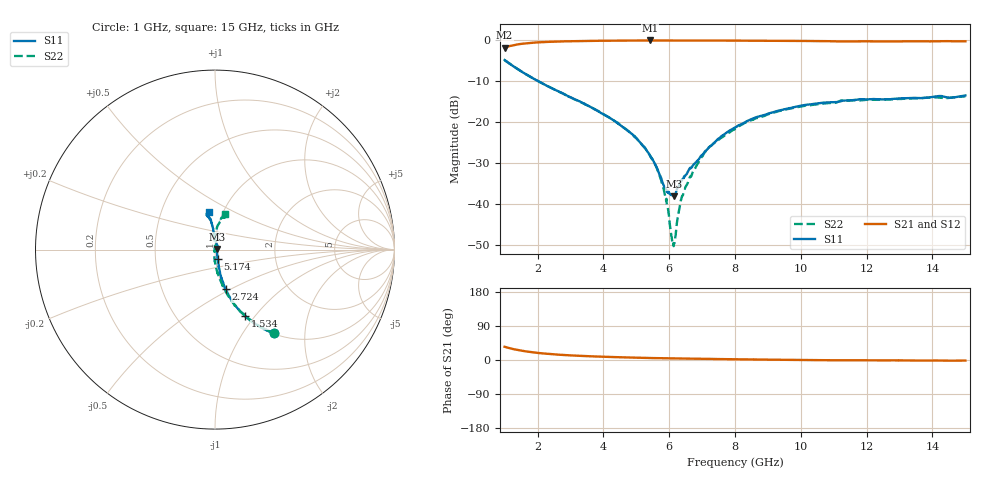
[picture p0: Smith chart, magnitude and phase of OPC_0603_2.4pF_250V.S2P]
! FILE NAME
! DATE 08/15/2012  09:51
! CORRECTED  DATA
# GHz  S  MA  R  50.00
!  FREQ  S11M  S11A  S21M  S21A  S12M  S12A  S22M  S22A
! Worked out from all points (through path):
!   1601 points, 1 GHz to 15 GHz, reference 50 ohm
!   highest |S21| = -0.06 dB at 5.419 GHz (marker M1); lowest = -1.8 dB at 1 GHz (marker M2)
!   group delay of S21, straight-line fit = 4.46 ps
!   lowest |S11| = -38.2 dB at 6.154 GHz (marker M3), VSWR 1.02, Z = 51.2 + j0.338 ohm
!   |S11| at or under -10 dB: 2.017 GHz to end of sweep
!   |S22| runs from -50.4 to -4.9 dB; largest |S21 - S12| = 0.0088
!   S11 on the Smith chart (normalised r, x): 1 GHz: 1.01, -1.40; 1.534 GHz: 1.01, -0.90; 2.724 GHz: 1.02, -0.47; 5.174 GHz: 1.02, -0.10; 15 GHz: 0.86, +0.37
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1  0.5719 -54.8  0.8126 34.9  0.8126 35.0  0.5716 -54.6
1.53375  0.4089 -65.5  0.9052 24.2  0.905 24.3  0.4086 -65.2
2.72375  0.2283 -74.9  0.9655 13.6  0.9657 13.7  0.2272 -76.4
3.33625  0.1735 -76.8  0.9775 10.8  0.9771 10.8  0.173 -80.0
4.3775  0.1007 -77.7  0.9887 7.5  0.9883 7.6  0.1007 -86.9
5.17375  0.05256 -73.6  0.9924 5.7  0.9916 5.7  0.05252 -92.7
5.41875  0.03885 -70.4  0.9933 5.2  0.9922 5.3  0.03839 -96.0
5.6725  0.02451 -61.8  0.9926 4.7  0.9922 4.8  0.02393 -100.6
5.9  0.01513 -35.7  0.9912 4.3  0.9903 4.4  0.01134 -107.6
6.08375  0.01285 2.1  0.9893 4.1  0.9891 4.1  0.003658 -140.0
6.15375  0.01233 15.5  0.9893 4.0  0.9887 4.0  0.003267 151.8
6.3025  0.01695 40.8  0.9881 3.8  0.9874 3.8  0.008435 95.2
6.39  0.01966 48.0  0.9871 3.8  0.9867 3.8  0.01234 90.4
6.5475  0.02365 58.8  0.9868 3.7  0.9866 3.7  0.01733 89.2
6.78375  0.03127 70.8  0.9885 3.5  0.9882 3.5  0.02696 92.8
7.23875  0.05026 85.4  0.9905 2.9  0.9903 2.9  0.04975 91.3
8  0.08551 93.3  0.9883 1.9  0.9877 1.9  0.08224 90.3
9.05  0.128 96.0  0.9836 0.9  0.9825 0.9  0.1258 84.9
10.33625  0.1649 98.0  0.9775 -0.2  0.977 -0.2  0.1612 78.8
11.26375  0.1812 100.9  0.9669 -0.6  0.9668 -0.6  0.1833 76.8
12.6725  0.1891 102.5  0.9632 -0.9  0.9633 -0.9  0.1883 73.7
15  0.2114 99.5  0.9702 -1.4  0.9697 -1.5  0.2067 74.0
